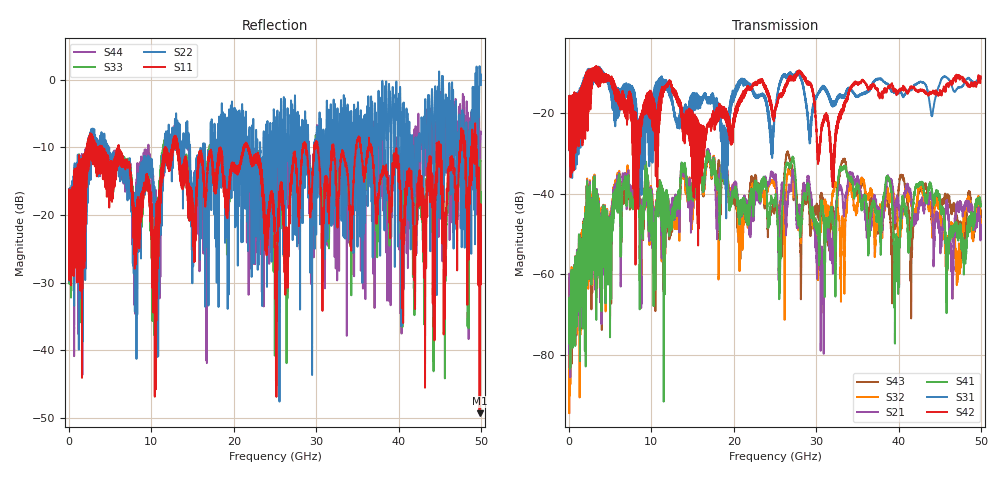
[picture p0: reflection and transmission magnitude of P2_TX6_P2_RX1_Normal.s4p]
!Keysight Technologies,N5225B,MY57041031,A.13.20.10
!Date: Friday, May 31, 2019 11:27:51
!Correction: S11(Full 4 Port(1,2,3,4))
!S12(Full 4 Port(1,2,3,4))
!S13(Full 4 Port(1,2,3,4))
!S14(Full 4 Port(1,2,3,4))
!S21(Full 4 Port(1,2,3,4))
!S22(Full 4 Port(1,2,3,4))
!S23(Full 4 Port(1,2,3,4))
!S24(Full 4 Port(1,2,3,4))
!S31(Full 4 Port(1,2,3,4))
!S32(Full 4 Port(1,2,3,4))
!S33(Full 4 Port(1,2,3,4))
!S34(Full 4 Port(1,2,3,4))
!S41(Full 4 Port(1,2,3,4))
!S42(Full 4 Port(1,2,3,4))
!S43(Full 4 Port(1,2,3,4))
!S44(Full 4 Port(1,2,3,4))
!S4P File: Measurements: <S11,S12,S13,S14>,
!<S21,S22,S23,S24>,
!<S31,S32,S33,S34>,
!<S41,S42,S43,S44>:
# Hz S  dB  R 50.0
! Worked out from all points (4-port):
!   5000 points, 10 MHz to 50 GHz, reference 50 ohm
!   strongest paths, dB at 10 MHz, 12.51 GHz, 25.01 GHz, 37.51 GHz, 50 GHz:
!     S42: -19.4, -14.1, -20.2, -14.5, -10.9
!     S31: -19.3, -16.8, -19.9, -11.6, -11.4
!     S41: -65.9, -46.4, -42.0, -44.8, -43.0
!     S21: -59.9, -45.0, -36.3, -43.6, -49.4
!     S32: -61.8, -45.4, -38.1, -44.1, -50.4
!     S43: -61.0, -47.5, -43.5, -48.9, -44.1
!   lowest |S11| = -49.4 dB at 49.84 GHz (marker M1), VSWR 1.01, Z = 50.1 - j0.337 ohm
!   |S11| at or under -10 dB: 6.028 GHz to 11.67 GHz (5.641 GHz wide, 63.8 % of centre); 21.74 GHz to 28.38 GHz (6.638 GHz wide, 26.5 % of centre); 36.76 GHz to 44.63 GHz (7.866 GHz wide, 19.3 % of centre)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
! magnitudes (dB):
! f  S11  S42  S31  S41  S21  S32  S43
! 10 MHz  -19.4  -19.4  -19.3  -65.9  -59.9  -61.8  -61.0
! 8.26 GHz  -18.4  -31.9  -21.9  -38.1  -35.4  -34.0  -36.6
! 29.06 GHz  -13.2  -12.3  -22.3  -37.5  -35.5  -37.2  -40.9
! 30.73 GHz  -25.3  -23.0  -13.4  -42.1  -56.2  -44.7  -40.5
! 34.22 GHz  -23.6  -13.8  -14.0  -36.4  -35.3  -39.0  -37.2
! 49.84 GHz  -49.4  -10.9  -11.1  -40.8  -46.9  -43.7  -45.1
! 50 GHz  -22.7  -10.9  -11.4  -43.0  -49.4  -50.4  -44.1
